(* Logix 5000 AddOnInstructionDefinition export T2MOV; software revision 32.02 *)

TYPE Exlar_Control :   // Tritex II Control
STRUCT
   EnableOutputs : INT;   // EnableOutputs
   InputEventsMode : INT;   // 4316
   InputEventsModeLevel : INT;   // 4318
   InputEventsMotion : INT;   // 4317
   HostCommandControlMode : INT;   // 4303
   HostPosition_low : INT;   // 4304
   HostPosition_high : INT;
   HostVelocity_low : INT;   // 4306
   HostVelocity_high : INT;
   HostAcceleration_low : INT;   // 4308
   HostAcceleration_high : INT;
   HostCurrent : INT;   // 4310
   InputEventsMoveEdge : INT;   // 4319
   JogSlowVelocity_low : INT;   // 6022
   JogSlowVelocity_high : INT;
   JogAcceleration_low : INT;   // 6026
   JogAcceleration_high : INT;
   MoveOption : INT;   // 6100
   MoveCurrentLimit : INT;   // 6101
   MoveAcceleration_low : INT;   // 6102
   MoveAcceleration_high : INT;
   MoveDeceleration_low : INT;   // 6500
   MoveDeceleration_high : INT;
   MovePrimaryOption : INT;   // 6106
   spare : INT;   // spare
   MovePrimaryPosition_low : INT;   // 6108
   MovePrimaryPosition_high : INT;
   MovePrimaryVelocity_low : INT;   // 6110
   MovePrimaryVelocity_high : INT;
   MoveSecondaryOption : INT;   // 6112
   spare2 : INT;   // spare
   MoveSecondaryPosition_low : INT;   // 6114
   MoveSecondaryPosition_high : INT;
   MoveSecondaryVelocity_low : INT;   // 6116
   MoveSecondaryVelocity_high : INT;
END_STRUCT
END_TYPE

TYPE Exlar_Drive :   // Tritex II Data
STRUCT
   Control : Exlar_Control;   // Control bits to send to the drive
   Status : Exlar_Status;   // Status bits received from the drive
END_STRUCT
END_TYPE

TYPE Exlar_Status :   // Tritex II Status
STRUCT
   EIP_Comm : INT;   // EIP module communication
   OutputEventsStatus : INT;   // 104
   OutputEventsMoveInPosition : INT;   // 108
   OutputEventsMotion : INT;   // 105
   OutputsEventsMotionActive : INT;   // 107
   PositionFeedback_low : INT;   // 378
   PositionFeedback_high : INT;
   SoftFaults : INT;   // 7
   HardFaults : INT;   // 6
   VelocityDisplay_low : INT;   // 356
   VelocityDisplay_high : INT;
   CurrentDisplay : INT;   // 567
   CurrentContinuous : INT;   // 565
   CurrentLimit : INT;   // 5108
   VoltageHallBattery : INT;   // 8
   VoltageBus : INT;   // 571
   TemperatureBoard : INT;   // 11
   TemperatureActuator : INT;   // 15
END_STRUCT
END_TYPE

ADD_ON_INSTRUCTION T2MOV   (* revision 1.1, vendor Exlar Corporation *)
// Help:
// Use the Tritex 2 Move (T2MOV) instruction to execute an drive move command
// The Move instruction is used to set up move profile parameters for both primary and secondary move.  The AOI also includes the ability to control the execution of the move.
// Configured for Exlar EIP AOI. 07/01/2014
// ----------------------------------------------------------------------------------------------------------------------------
// Parameters Bit Definition
// ----------------------------------------------------------------------------------------------------------------------------
// Execute:   (Input) Control Move 0 commands
// ------------------------------------------------------------------
//      Execute.0:     Move 0 Maintained
//      Execute.1:     Move 0 Momentary
// Options:   (Input) Move 0 Options
// ------------------------------------------------------------------
//      Options.0:     Secondary Motion Enable
// PrimOption:   (Input) Move 0 Primary Options
// ------------------------------------------------------------------
//      PrimOption.2.1.0:    Three bits determine Primary Move Options
//                                     %000 = Absolute Position
//                                     %001 = Incremental
//                                     %010 = Unlimited(+)
//                                     %011 = Unlimted(-)
//                                     %100 = Absolute(+) only
//                                     %101 = Absolute(-) only
//      PrimOption.3:     Limit maximum Current
//      PrimOption.4:     Terminate on Current Limit
//      PrimOption.5:     Fault if terminated by current limit
// SecOption:   (Input) Move 0 Secondary Options
// ------------------------------------------------------------------
//      SecOption.2.1.0:    Three bits determine Secondary Move Options
//                                     %000 = Absolute Position
//                                     %001 = Incremental
//                                     %010 = Unlimited(+)
//                                     %011 = Unlimted(-)
//                                     %100 = Absolute(+) only
//                                     %101 = Absolute(-) only
//      SecOption.3:     Limit maximum Current
//      SecOption.4:     Terminate on Current Limit
//      SecOption.5:     Fault if terminated by current limit
// Active:  (Output) Move 0 status information
// ------------------------------------------------------------------
//      Active.0:     Ready -  is set when both the ENABLED and HOMED flags are active.
//      Active.1:     Move 0 in Position
//      Active.2:     Move 0 active
VAR_IN_OUT
   Drive : Exlar_Drive; {required}   // Drive
   Units : REAL[5]; {required}   // Units
END_VAR
VAR_INPUT
   Execute : INT; {visible}   // Move Control
        .0   // Maintained
        .1   // Momentary
   Options : INT; {visible}   // Move Options
        .0   // Secondary Motion Enable
   CurrentLimit : REAL; {visible}   // Move Current Limit
   Acceleration : INT; {visible}   // Acceleration rate of the drive in Accel Units
   Deceleration : INT; {visible}   // Deceleration rate of the drive in Accel Units
   Prim_Position : REAL; {visible}   // Absolute position or incremental distance for the move
   Prim_Velocity : REAL; {visible}   // Speed to move the drive in Speed Units
   Prim_Option : INT; {visible}   // Primary Move Options
        .0   // TYPE Bit
        .1   // TYPE Bit
        .2   // TYPE Bit
        .3   // Limit maximum Current
        .4   // Terminate on Current Limit
        .5   // Fault if terminated by current limit
   Sec_Position : REAL; {visible}   // Absolute position or incremental distance for the move
   Sec_Velocity : REAL; {visible}   // Speed to move the drive in Speed Units
   Sec_Option : INT; {visible}   // Secondary Move Options
        .0   // TYPE Bit
        .1   // TYPE Bit
        .2   // TYPE Bit
        .3   // Limit maximum Current
        .4   // Terminate on Current Limit
        .5   // Fault if terminated by current limit
END_VAR
VAR_OUTPUT
   DF : BOOL; {access Read Only, visible}   // A Drive Fault is active
   ER : BOOL; {access Read Only, visible}   // A Instruction error is Active
   IP : BOOL; {access Read Only, visible}   // Move 0 In Position
   Active : INT; {access Read Only, visible}   // Active
        .0   // Ready
        .1   // Move 0 In Position
        .2   // Move 0 active
END_VAR
VAR
   tempDINT : DINT; {access None}   // Temporary Register used in calculating units
END_VAR

ROUTINE Logic   (* structured text *)
   (***********************************************)
   (*   Exlar Tritex 2 Move                       *)
   (*                                             *)
   (***********************************************)
   (*
    Revision History
    -------
    3.7.2023   Fixed bug of array pointer for Modbus ID 6101 scaling
   
   *)
   
   (********** Inputs ***********)
   
   (* Execute *)
   	(* 4318.0  Move 0 Maintained *)
   	if Execute.0 then
   		Drive.Control.InputEventsModeLevel.0 := 1;
   	else
   		Drive.Control.InputEventsModeLevel.0 := 0;
   	end_if;
   
   	(* 4319.0  Move 0 Momentary *)
   	if Execute.1 then
   		Drive.Control.InputEventsMoveEdge.0 := 1;
   	else
   		Drive.Control.InputEventsMoveEdge.0 := 0;
   	end_if;
   
   (* Option *)
   	(* 6100.0  Secondary Motion Enable *)
   	if Options.0 then
   		Drive.Control.MoveOption.0 := 1;
   	else
   		Drive.Control.MoveOption.0 := 0;
   	end_if;
   
   (* Primary Option *)
   	(* 6106.0  - Move Type *)
   	if Prim_Option.0 then
   		Drive.Control.MovePrimaryOption.0 := 1;
   	else
   		Drive.Control.MovePrimaryOption.0 := 0;
   	end_if;
   	(* 6106.1  - Move Type *)
   	if Prim_Option.1 then
   		Drive.Control.MovePrimaryOption.1 := 1;
   	else
   		Drive.Control.MovePrimaryOption.1 := 0;
   	end_if;
   	(* 6106.2  - Move Type *)
   	if Prim_Option.2 then
   		Drive.Control.MovePrimaryOption.2 := 1;
   	else
   		Drive.Control.MovePrimaryOption.2 := 0;
   	end_if;
   
   	(* 6106.4 Limit maximum Current *)
   	if Prim_Option.3 then
   		Drive.Control.MovePrimaryOption.4 := 1;
   	else
   		Drive.Control.MovePrimaryOption.4 := 0;
   	end_if;
   
   	(* 6106.8 Terminate on Current Limit *)
   	if Prim_Option.4 then
   		Drive.Control.MovePrimaryOption.8 := 1;
   	else
   		Drive.Control.MovePrimaryOption.8 := 0;
   	end_if;
   
   	(* 6106.12 Fault if terminated by current limit *)
   	if Prim_Option.5 then
   		Drive.Control.MovePrimaryOption.12 := 1;
   	else
   		Drive.Control.MovePrimaryOption.12 := 0;
   	end_if;
   
   (* Secondary Option	*)
   	(* 6112.0  - Move Type *)
   	if Sec_Option.0 then
   		Drive.Control.MoveSecondaryOption.0:= 1;
   	else
   		Drive.Control.MoveSecondaryOption.0	:= 0;
   	end_if;
   
   	(* 6112.1  - Move Type *)
   	if Sec_Option.1 then
   		Drive.Control.MoveSecondaryOption.1	 := 1;
   	else
   		Drive.Control.MoveSecondaryOption.1	 := 0;
   	end_if;
   
   	(* 6112.2  - Move Type *)
   	if Sec_Option.2 then
   		Drive.Control.MoveSecondaryOption.2	 := 1;
   	else
   		Drive.Control.MoveSecondaryOption.2	 := 0;
   	end_if;
   
   	(* 6112.4 Limit maximum Current *)
   	if Sec_Option.3 then
   		Drive.Control.MoveSecondaryOption.4	 := 1;
   	else
   		Drive.Control.MoveSecondaryOption.4	 := 0;
   	end_if;
   
   	(* 6112.8 Terminate on Current Limit *)
   	if Sec_Option.4 then
   		Drive.Control.MoveSecondaryOption.8	 := 1;
   	else
   		Drive.Control.MoveSecondaryOption.8	 := 0;
   	end_if;
   
   	(* 6112.12 Fault if terminated by current limit *)
   	if Sec_Option.5 then
   		Drive.Control.MoveSecondaryOption.12	 := 1;
   	else
   		Drive.Control.MoveSecondaryOption.12	 := 0;
   	end_if;
   
   
   (********** Outputs **********)
   (* Drive Faults Active *)
   	(* 104.03 Fault *)
   	If Drive.Status.OutputEventsStatus.3 then
    		DF := 1;
   	Else
   		DF := 0;
   	End_If;
   
   (* Active *)
   	(* 104.2 Ready *)
   	If Drive.Status.OutputEventsStatus.2 Then
   		Active.0 := 1;
   	else
   		Active.0 := 0;
   	end_if;
   
   	(* 108.0 Move 0 in Position *)
   	If Drive.Status.OutputEventsMoveInPosition.0 Then
   		Active.1 := 1;
   		IP := 1;
   	else
   		Active.1 := 0;
   		IP := 0;
   	end_if;
   
   	(* 107.0 Move 0 Moving *)
   	If Drive.Status.OutputsEventsMotionActive.0 Then
   		Active.2 := 1;
   	else
   		Active.2 := 0;
   	end_if;
   
   
   (* Convert Units *)
   	IF Units[0] = 0 THEN
   		ER	:= 1;
   	else
   		ER  := 0;
   
   		(** Move Group **)
   	 	(* ID:6102, Move.0.Acceleration:  ModuleOutputs[20],ModuleOutputs[19] *)
   		tempDINT := Acceleration / Units[3];
   		cps(tempDINT, Drive.Control.MoveAcceleration_low,2);
   
   		(* ID:6500, Move.0.Deceleration:  ModuleOutputs[22],ModuleOutputs[21] *)
   		tempDINT := Deceleration / Units[3];
   		cps(tempDINT, Drive.Control.MoveDeceleration_low,2);
   
   		(* Primary Group **)
   		(* ID:6110, Move.0.Primary.Velocity:  ModuleOutputs[28],ModuleOutputs[27] *)
   		tempDINT := Prim_Velocity / Units[2];
   		cps(tempDINT, Drive.Control.MovePrimaryVelocity_low,2);
   
   		(* Secondary Group **)
   		(* ID:6116, Move.0.Secondary.Velocity:  ModuleOutputs[34],ModuleOutputs[33] *)
   		tempDINT := Sec_Velocity / Units[2];
   		cps(tempDINT, Drive.Control.MoveSecondaryVelocity_low,2);
   
   		(* ID:6114, Move.0.Secondary.Position:  ModuleOutputs[32],ModuleOutputs[31] *)
   		tempDINT := Sec_Position / Units[1];
   		cps(tempDINT, Drive.Control.MoveSecondaryPosition_low,2);
   
   		(* ID:6108, Move.0.Primary.Position:  ModuleOutputs[26],ModuleOutputs[25] *)
   		tempDINT := Prim_Position / Units[1];
   		cps(tempDINT, Drive.Control.MovePrimaryPosition_low,2);
   
   
   		(* Current Scale   *)
   		(*       0: AMPs   *)
   		(*       1: %      *)
   		(* ID:6101,  Move.0.CurrentLimit:  ModuleOutputs[18] *)
   		if Units[4] = 0	then
   			Drive.Control.MoveCurrentLimit := CurrentLimit / 0.0078125 ;
   		else
   			(* Use for % ,ID:5108, Config.CurrentLimit:   ModuleInputs[13],  *)
   			Drive.Control.MoveCurrentLimit := Drive.Status.CurrentLimit * (CurrentLimit /100);
   		end_if;
   	end_if;
   
   
   
   
   
   
   
   
   
   
END_ROUTINE
END_ADD_ON_INSTRUCTION
